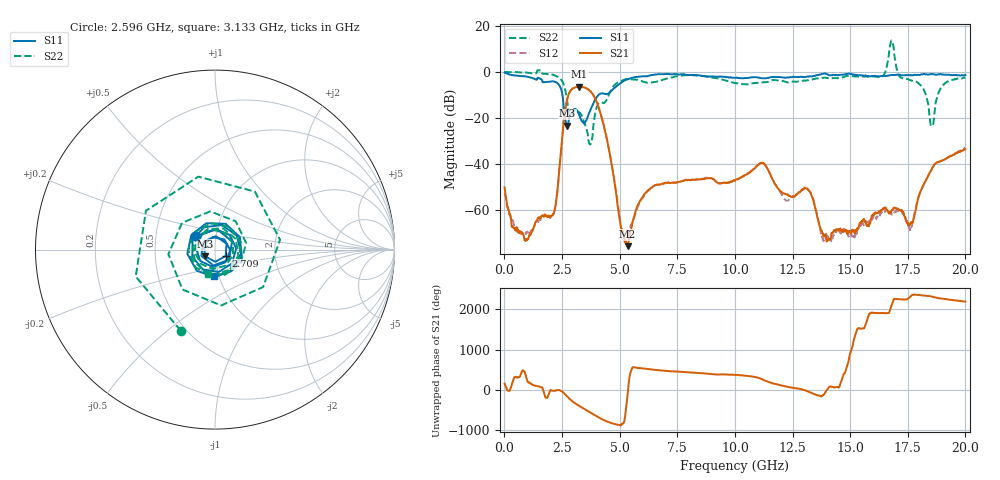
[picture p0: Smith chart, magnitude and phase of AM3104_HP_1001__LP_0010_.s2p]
!Created with skrf (http://scikit-rf.org).
# Hz S RI R 50.0
!freq ReS11 ImS11 ReS21 ImS21 ReS12 ImS12 ReS22 ImS22
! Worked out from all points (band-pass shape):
!   1601 points, 10 MHz to 20 GHz, reference 50 ohm
!   highest |S21| = -6.44 dB at 3.246 GHz (marker M1); lowest = -76.0 dB at 5.345 GHz (marker M2)
!   |S21| within 3 dB of the highest: 2.801 GHz to 3.815 GHz (1.014 GHz wide, 30.6 % of centre)
!   lowest |S11| = -23.5 dB at 2.734 GHz (marker M3), VSWR 1.14, Z = 44.6 - j3.34 ohm
!   |S11| at or under -10 dB: 2.518 GHz to 4.084 GHz (1.566 GHz wide, 47.4 % of centre)
!   |S22| runs from -31.6 to 13.7 dB; largest |S21 - S12| = 0.025
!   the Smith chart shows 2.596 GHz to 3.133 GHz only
!   S11 on the Smith chart (normalised r, x): 2.596 GHz: 0.80, +0.12; 2.709 GHz: 1.12, -0.08; 3.133 GHz: 0.94, -0.29
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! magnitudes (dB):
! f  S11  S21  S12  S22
! 10 MHz  -0.3  -50.3  -52.9  0.0
! 934.5 MHz  -2.0  -73.0  -70.7  -0.2
! 2.071 GHz  -4.1  -62.4  -63.3  -1.2
! 2.596 GHz  -17.6  -20.2  -20.2  -6.2
! 2.709 GHz  -23.1  -12.7  -12.7  -11.7
! 2.734 GHz  -23.5  -11.6  -11.6  -13.4
! 3.133 GHz  -16.5  -6.6  -6.6  -16.8
! 3.246 GHz  -18.8  -6.4  -6.5  -17.7
! 3.346 GHz  -21.2  -6.5  -6.6  -18.8
! 3.733 GHz  -16.7  -8.4  -8.5  -31.6
! 4.17 GHz  -9.5  -18.0  -18.0  -13.4
! 5.345 GHz  -3.2  -76.0  -71.3  -3.1
! 6.682 GHz  -1.0  -49.2  -49.2  -4.1
! 10.01 GHz  -2.7  -47.5  -47.2  -4.8
! 11.19 GHz  -2.8  -39.7  -39.7  -4.6
! 13.34 GHz  -2.0  -54.3  -54.0  -3.3
! 13.83 GHz  -0.9  -71.1  -72.9  -2.7
! 16.68 GHz  -1.5  -61.7  -61.5  7.2
! 17.63 GHz  -1.4  -65.7  -67.7  -3.6
! 18.54 GHz  -0.9  -42.3  -42.4  -23.6
! 19 GHz  -1.2  -38.6  -38.7  -6.2
! 20 GHz  -1.4  -33.8  -33.1  -2.5
